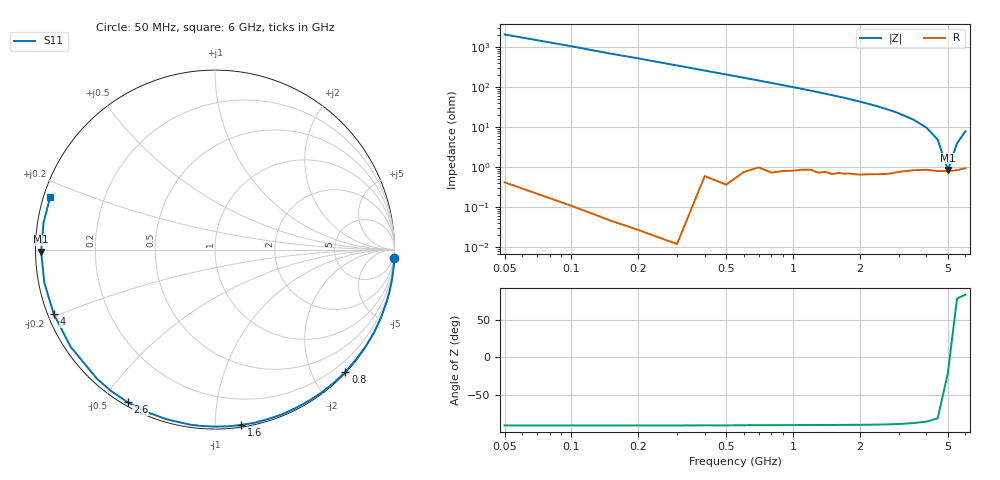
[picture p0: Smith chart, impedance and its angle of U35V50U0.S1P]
! SIEMENS Discrete & RF Semiconductors
! BBY53-02W
! Si Tuning Diode in SCD-80
! VR = 5.5 V
! S-Parameters:  September  1997
# GHz  S  MA  R  50
!  f  S11
! GHz  MAG  ANG
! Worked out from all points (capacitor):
!   34 points, 50 MHz to 6 GHz, reference 50 ohm
!   read as one part to ground: C = 1.56 pF near 50 MHz
!   lowest |Z| = 853 mohm at 5 GHz (marker M1)
!   series resonance near 5.037 GHz, so ESL is about 640 pH
!   S11 on the Smith chart (normalised r, x): 50 MHz: 0, -41; 800 MHz: 0.01, -2.53; 1.6 GHz: 0.01, -1.16; 2.6 GHz: 0.01, -0.58; 4 GHz: 0.02, -0.19; 6 GHz: 0.02, +0.16
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0.05  1 -2.8
0.2  1 -11.0
0.3  1 -16.5
0.4  0.9991 -22.0
0.5  0.9992 -27.4
0.6  0.9976 -32.7
0.8  0.996 -43.2
0.9  0.9946 -48.4
1  0.9935 -53.3
1.1  0.9918 -58.3
1.2  0.9906 -63.1
1.3  0.9909 -67.9
1.4  0.9893 -72.6
1.5  0.9896 -77.2
1.6  0.9879 -81.5
1.8  0.9862 -90.1
2  0.9852 -98.1
2.2  0.9832 -105.8
2.4  0.9816 -113.0
2.6  0.9801 -119.8
2.8  0.9779 -126.3
3  0.9749 -132.3
3.5  0.9698 -146.0
4  0.9674 -158.1
4.5  0.9688 -169.0
5  0.9686 -179.3
5.5  0.9671 171.2
6  0.964 162.3
